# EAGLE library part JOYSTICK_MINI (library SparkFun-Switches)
Small Tactile Joystick w/ Select Switch A 5-way tactile switch allows for a joystick-like interface in a very small package. Part #: 4UCON SF303GJ26 SparkFun Products 5-way Tactile Switch (COM-10063) Used on SparkFun Block for Intel® Edison - OLED (DEV-13035) Used on CAN-BUS Shield (DEV-13262)
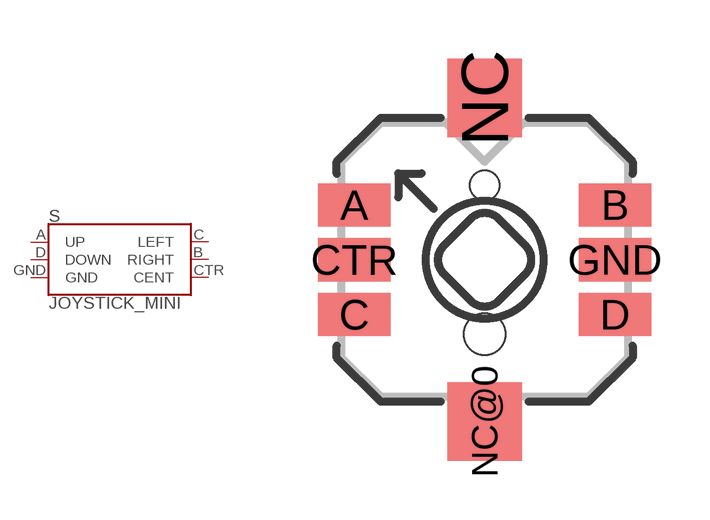
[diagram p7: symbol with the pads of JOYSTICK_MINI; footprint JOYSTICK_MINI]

Designator prefix S

## JOYSTICK_MINI (PROD_ID: SWCH-09905; SF_SKU: COM-10063)  [JOYSTICK_MINI]
A  UP
B  RIGHT
C  LEFT
CTR  CENT
D  DOWN
GND  GND

## Footprint JOYSTICK_MINI (pad centres in mm)
Small Tactile Joystick w/ Select Switch A 5-way tactile switch allows for a joystick-like interface in a very small package. Datasheet
smd 1.85 x 1.1: A -3.325,1.4; B 3.325,1.4; C -3.325,-1.4; CTR -3.325,0; D 3.325,-1.4; GND 3.325,0
smd 1.9 x 2: NC 0,4.13; NC@0 0,-4.13
hole 0.75 at 0,1.9
hole 1.05 at 0,-1.9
